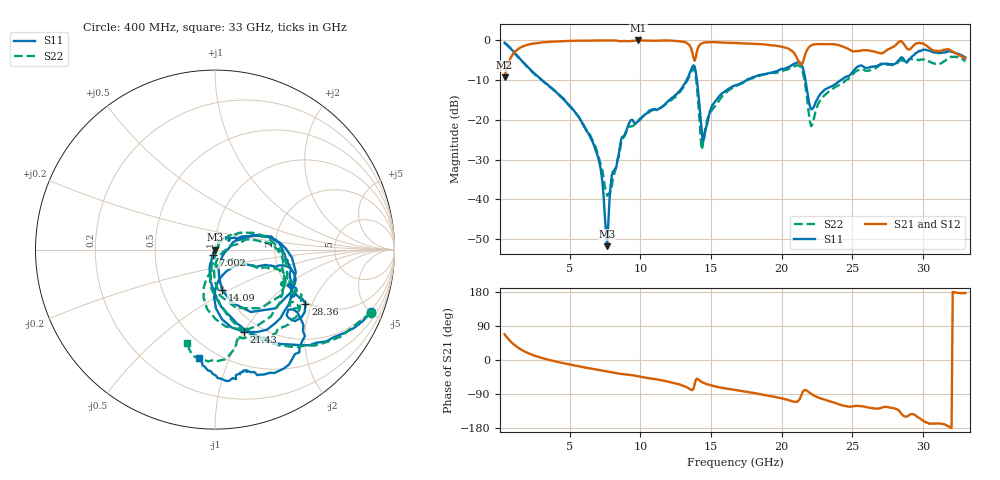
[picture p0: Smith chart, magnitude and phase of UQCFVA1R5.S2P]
!  Part Number  UQCFVA1R5  Mounting Orientation: Horizontal
!  Description: Ultra Low ESR Microwave capacitors
!  Application: Coupling, Bypass, Tuning, DC Block
!  Filters, Matching
# GHZ S DB R 50
! Freq  |S11|  S11 Ph  |S21|  S21 Ph  |S12|  S12 Ph  |S22|  S22 Ph
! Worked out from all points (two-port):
!   401 points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, 400 MHz to 33 GHz, reference 50 ohm
!   highest |S21| = 0.00 dB at 9.854 GHz (marker M1); lowest = -9.3 dB at 400 MHz (marker M2)
!   |S21| within 3 dB of the highest: 1.092 GHz to 13.68 GHz (12.59 GHz wide, 170 % of centre); 13.99 GHz to 20.84 GHz (6.85 GHz wide, 39.3 % of centre)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
!   lowest |S11| = -51.8 dB at 7.654 GHz (marker M3), VSWR 1.01, Z = 50.3 - j0.0279 ohm
!   |S11| at or under -10 dB: 3.053 GHz to 13.28 GHz (10.23 GHz wide, 125 % of centre); 14 GHz to 17.5 GHz (3.494 GHz wide, 22.2 % of centre); 21.69 GHz to 24.18 GHz (2.49 GHz wide, 10.9 % of centre)
!   |S22| runs from -39.1 to -0.6 dB; largest |S21 - S12| = 0.015
!   S11 on the Smith chart (normalised r, x): 400 MHz: 0.89, -5.03; 7.002 GHz: 0.97, -0.06; 14.09 GHz: 0.97, -0.46; 21.43 GHz: 0.84, -1.01; 28.36 GHz: 1.95, -1.79; 33 GHz: 0.41, -0.78
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0.4  -0.57 -21.9  -9.26 67.9  -9.27 67.8  -0.56 -22.1
2.193  -7.24 -73.0  -0.95 16.1  -0.96 15.7  -7.32 -74.4
5.861  -20.56 -107.8  -0.05 -18.2  -0.04 -18.2  -20.50 -101.6
7.002  -29.33 -112.2  -0.01 -25.9  -0.02 -25.9  -28.60 -92.5
7.654  -51.80 -6.2  -0.01 -30.3  0.00 -30.3  -39.11 -37.1
8.061  -33.05 36.7  -0.02 -32.9  -0.02 -32.9  -34.97 31.8
8.713  -24.28 56.0  -0.16 -36.6  -0.16 -36.6  -24.91 55.9
9.854  -20.31 36.3  0.00 -42.9  -0.01 -42.9  -20.21 45.9
11.321  -17.18 24.9  -0.03 -52.1  -0.04 -52.0  -17.20 37.1
13.114  -11.03 15.7  -0.42 -68.9  -0.44 -68.8  -11.43 17.7
13.685  -6.61 -15.6  -3.07 -79.4  -3.07 -79.3  -7.28 -21.2
14.092  -12.85 -80.1  -1.77 -50.8  -1.82 -51.1  -15.22 -90.8
14.5  -24.86 -14.7  -0.56 -60.7  -0.57 -60.6  -24.16 -0.6
16.7  -11.33 15.5  -0.61 -79.0  -0.63 -78.8  -11.62 9.6
20.449  -6.76 -22.6  -2.01 -105.2  -2.09 -105.1  -7.30 -29.2
21.427  -6.27 -70.4  -5.98 -89.8  -6.02 -90.0  -7.29 -82.3
22.161  -17.29 -51.7  -1.10 -91.0  -1.12 -91.1  -21.28 -51.8
24.198  -9.94 -16.3  -1.36 -118.8  -1.36 -118.5  -11.07 -21.8
27.621  -6.06 -31.5  -2.13 -125.4  -2.08 -125.2  -6.02 -29.7
28.355  -4.63 -30.9  -0.24 -135.8  -0.24 -136.2  -5.12 -30.3
30.311  -2.48 -65.9  -1.46 -165.4  -1.46 -165.6  -5.15 -65.0
33  -4.30 -98.2  -4.51 176.8  -4.46 177.1  -5.27 -106.4
